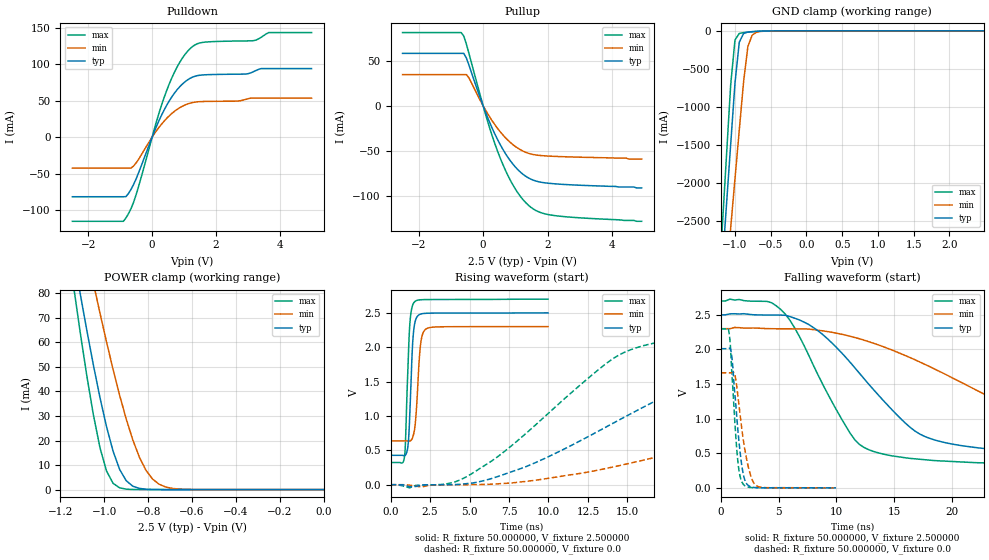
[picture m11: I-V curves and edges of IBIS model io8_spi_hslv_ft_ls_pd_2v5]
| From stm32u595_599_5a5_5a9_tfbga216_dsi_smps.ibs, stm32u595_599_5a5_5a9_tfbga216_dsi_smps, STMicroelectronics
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|   Model io8_spi_hslv_ft_ls_pd_2v5
[Model]  io8_spi_hslv_ft_ls_pd_2v5
Model_type I/O
Polarity   Non-Inverting
Enable   Active-Low
Vinl =   0.750000V
Vinh =   1.750000V
Vmeas =  1.250000V
Cref =   50.000000pF
Rref =   100.000000M
Vref =   0.0V
C_comp   3.438200pF   3.436700pF   3.473300pF
[Temperature Range]   25.000000   0.140000k   -40.000000
[Pullup Reference]   2.500000V   2.300000V   2.700000V
[Pulldown Reference]   0.0V   0.0V   0.0V
[POWER Clamp Reference]   2.500000V   2.300000V   2.700000V
[GND Clamp Reference]   0.0V   0.0V   0.0V
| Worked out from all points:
|   slope of the pulldown table from 0 to 0.375 V, typ, clamps not added: 10.1 ohm
|   slope of the pullup table from 0 to 0.375 V, typ, clamps not added: 11.7 ohm
|   GND clamp passes 1 mA (typ) near -0.50 V on its own axis
|   POWER clamp passes 1 mA (typ) near -0.86 V on its own axis
|   rising waveform, R_fixture 50.000000, V_fixture 2.500000: 20-80 % time 223ps typ, 270ps min, 220ps max; typ from 0.427 V to 2.5 V
|   rising waveform, R_fixture 50.000000, V_fixture 0.0: 20-80 % time 10.5ns typ, 19ns min, 7.04ns max; typ from 0 V to 2.01 V
|   falling waveform, R_fixture 50.000000, V_fixture 2.500000: 20-80 % time 6.96ns typ, 13.6ns min, 4.48ns max; typ from 2.5 V to 0.427 V
|   falling waveform, R_fixture 50.000000, V_fixture 0.0: 20-80 % time 653ps typ, 861ps min, 533ps max; typ from 2.01 V to 0 V
[Pulldown]
|Voltage   I(typ)   I(min)   I(max)
-2.5V     -81.62mA   -42.31mA   -115.3mA
-900mV    -81.62mA   -42.31mA   -115.3mA
-820mV    -81.42mA   -42.31mA   -110.6mA
-500mV    -56.95mA   -35.08mA   -78.57mA
140mV     15.18mA    9.02mA     22.02mA
460mV     44mA       25.98mA    64.37mA
860mV     68.91mA    40.27mA    102.2mA
1.26V     82.21mA    47.42mA    124mA
1.66V     85.53mA    48.99mA    130.3mA
3.18V     89.84mA    53.65mA    132.3mA
3.66V     94.05mA    53.65mA    143.4mA
5V        94.05mA    53.65mA    143.4mA
[Pullup]
|Voltage   I(typ)   I(min)   I(max)
-2.5V     58.05mA    34.52mA    81.07mA
-680mV    58.05mA    34.52mA    81.07mA
-600mV    58.05mA    34.52mA    77.18mA
-440mV    45.11mA    30.86mA    58.07mA
120mV     -11.17mA   -7.509mA   -14.95mA
520mV     -42.32mA   -28.36mA   -56.93mA
760mV     -56.64mA   -37.85mA   -76.55mA
1V        -67.83mA   -45.13mA   -92.22mA
1.48V     -81.29mA   -53.4mA    -112.4mA
1.8V      -84.73mA   -55.19mA   -118.5mA
2.28V     -86.63mA   -56.16mA   -121.9mA
4.92V     -91mA      -59mA      -128mA
[GND_clamp]
|Voltage   I(typ)   I(min)   I(max)
-2.5V     -9.641A    -9.693A    -9.352A
-1.18V    -3.114A    -3.874A    -2.614A
-1.12V    -2.301A    -3.23A     -1.656A
-1.06V    -1.489A    -2.587A    -706.2mA
-1V       -685.8mA   -1.945A    -119.3mA
-940mV    -149.8mA   -1.304A    -34.74mA
-880mV    -35.55mA   -672.6mA   -23.08mA
-820mV    -16.2mA    -206.4mA   -17.29mA
-760mV    -10.59mA   -57.56mA   -12.42mA
-700mV    -7.162mA   -18.75mA   -8.254mA
-400mV    -112.4uA   -385.2uA   -53.46uA
2.48V     63.1uA     48.03uA    77.39uA
[POWER_clamp]
|Voltage   I(typ)   I(min)   I(max)
-2.49V    881mA      773.1mA    1.07A
-1.14V    95.25mA    122.7mA    82.82mA
-1.11V    79.9mA     109.7mA    64.14mA
-1.05V    50.87mA    84.26mA    30.57mA
-1.02V    37.63mA    72.04mA    17.17mA
-990mV    25.71mA    60.25mA    7.621mA
-930mV    8.217mA    38.43mA    713.9uA
-900mV    3.624mA    28.77mA    182.8uA
-840mV    490.7uA    13.24mA    11.35uA
-780mV    56.55uA    4.324mA    699nA
-660mV    716.7nA    226uA      9.786nA
0V        0A         19.53nA    0A
[Ramp]
| variable   typ   min   max
dV/dt_r  1.20630/10.50631n   0.99744/18.94632n   1.37748/7.02026n
dV/dt_f  1.24320/6.95214n   0.99724/13.55268n   1.42604/4.46674n
R_load = 50.000000
[Rising Waveform]
R_fixture= 50.000000
V_fixture= 2.500000
V_fixture_min= 2.300000
V_fixture_max= 2.700000
|time   V(typ)   V(min)   V(max)
0s        427.5mV    637.3mV    322.7mV
880.9ps   422.8mV    637.4mV    408.4mV
940.9ps   431.1mV    637.3mV    606.4mV
1.081ns   530.9mV    635.3mV    1.584V
1.201ns   938.3mV    633.7mV    2.273V
1.381ns   1.988V     677.8mV    2.6V
1.522ns   2.337V     809mV      2.661V
1.882ns   2.48V      2.003V     2.69V
2.222ns   2.493V     2.261V     2.693V
9.97ns    2.499V     2.299V     2.699V
[Rising Waveform]
R_fixture= 50.000000
V_fixture= 0.0
V_fixture_min= 0.0
V_fixture_max= 0.0
|time   V(typ)   V(min)   V(max)
0s        2.072nV    118.4nV    2.101nV
4.805ns   15.14mV    -15.62uV   115mV
8.809ns   284.6mV    54.82mV    793.2mV
13.61ns   835.3mV    234.7mV    1.756V
15.22ns   1.032V     315.3mV    1.965V
20.42ns   1.605V     603.7mV    2.181V
24.42ns   1.802V     832.8mV    2.238V
37.24ns   1.967V     1.407V     2.289V
57.26ns   2.006V     1.607V     2.296V
199.4ns   2.01V      1.663V     2.296V
[Falling Waveform]
R_fixture= 50.000000
V_fixture= 2.500000
V_fixture_min= 2.300000
V_fixture_max= 2.700000
|time   V(typ)   V(min)   V(max)
0s        2.499V     2.299V     2.699V
4.404ns   2.497V     2.299V     2.674V
6.006ns   2.473V     2.297V     2.415V
7.608ns   2.36V      2.294V     1.917V
12.01ns   1.653V     2.153V     625.4mV
16.02ns   927.5mV    1.907V     433.1mV
18.42ns   695.7mV    1.723V     394.9mV
29.23ns   495.7mV    951.7mV    338.3mV
46.85ns   442.1mV    723.3mV    324.8mV
199.4ns   427.5mV    637.3mV    322.7mV
[Falling Waveform]
R_fixture= 50.000000
V_fixture= 0.0
V_fixture_min= 0.0
V_fixture_max= 0.0
|time   V(typ)   V(min)   V(max)
0s        2.01V      1.663V     2.296V
660.7ps   2.011V     1.663V     2.294V
800.8ps   2.019V     1.663V     2.133V
900.9ps   1.964V     1.662V     1.858V
1.201ns   1.396V     1.647V     1.01V
1.461ns   880.3mV    1.365V     421.7mV
1.942ns   206.3mV    708.1mV    54.31mV
2.563ns   17.57mV    193mV      5.635mV
3.123ns   2.716mV    27.19mV    2.031mV
9.97ns    2.072nV    118.4nV    2.101nV
